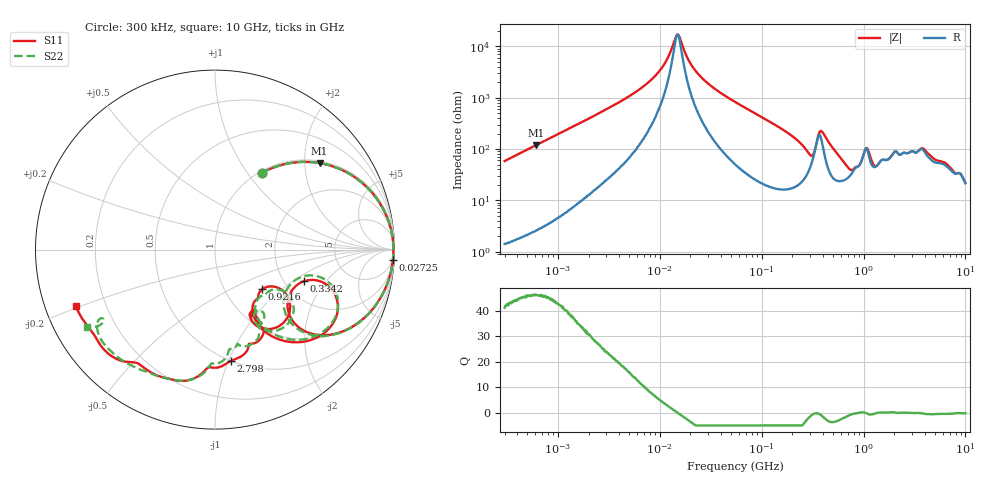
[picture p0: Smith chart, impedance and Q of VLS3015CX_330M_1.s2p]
! S-Parameter Data Generated by TDK Corporation
! Copyright(C) 2020 TDK Corporation.
! All Rights Reserved.
! TDK P/N: VLS3015CX-330M-1 (Inductor)
! Property: L=33uH at 1MHz
! Size(LxWxT): 3x3x1.5mm
! Model Type: s2p (Touchstone File Format Version 1.0)
! Frequency: DC=Yes Start=0.3MHz Stop=10000MHz 802points Log-sweep
! Model Generated on Aug. 18, 2020
! Port Assignments:
!  1 ---@@@--- 2
! Applicable Conditions:
!  Temperature = 25 degC
!  DC Bias Current = 0 A
!  Small Signal Operation
! Terms and conditions regarding TDK Simulation Models
! (1)This simulation model is being provided solely for informational purposes. Please refer to the specifications of the products in terms of detailed characteristics of such products.
! (2)In no event shall TDK Corporation of any of its subsidiaries be liable for any loss or damage arising, directly or indirectly,
!  From any information contained in this simulation model, including, but not limited to loss or damages arising from any inaccuracies, omissions or errors in connection with such information.
! (3)Any and all copyrights on this simulation model are owned by TDK Corporation.
!  Duplication or redistribution of this simulation model without prior written permission from TDK Corporation is prohibited.
! (4)This simulation model is subject to any modification or change without any prior notice.
! (5)Neither TDK Corporation nor any of its subsidiaries shall make any warranty, express or implied,
!  Including but not limited to the correctness, implied warranties of merchantability and fitness for a particular purpose with respect to this simulation models.
! (6)The use of this simulation model shall be deemed to have consented to the terms and conditions hereof.
# Hz S MA R 50
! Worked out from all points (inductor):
!   801 points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, 300 kHz to 10 GHz, reference 50 ohm
!   read as one part in series: L = 31 uH near 318.3 kHz
!   highest Q = 46.2 at 610.3 kHz (marker M1), where L = 30.9 uH
!   self-resonance near 14.9 MHz
!   S11 on the Smith chart (normalised r, x): 300 kHz: 1.03, +1.17; 27.25 MHz: 4, -34; 334.2 MHz: 2.53, -1.23; 921.6 MHz: 1.49, -0.75; 2.798 GHz: 0.50, -1.02; 10 GHz: 0.09, -0.19
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300000  0.4998 58.7  0.8544 -29.9  0.8538 -29.9  0.4991 58.7
610333  0.7562 39.6  0.6373 -49.2  0.6374 -49.1  0.7564 39.6
1713600  0.9499 16.5  0.285 -71.8  0.285 -71.8  0.9501 16.5
9671944  0.9937 1.5  0.03187 -78.1  0.03185 -78.1  0.9937 1.5
1.49005e7  0.9941 -0.4  0.005795 -3.4  0.005776 -3.5  0.9942 -0.4
2.036513e7  0.9938 -1.8  0.02258 73.3  0.02256 73.3  0.9938 -1.8
2.725275e7  0.9929 -3.3  0.04479 79.1  0.04477 79.1  0.9929 -3.3
5.477226e7  0.9856 -8.3  0.1184 78.2  0.1184 78.2  0.9857 -8.3
1.291483e8  0.9391 -20.6  0.296 66.1  0.2959 66.1  0.9389 -20.8
2.22675e8  0.7992 -36.4  0.5119 46.3  0.5118 46.3  0.7969 -36.9
3.126428e8  0.4887 -33.0  0.6014 10.8  0.6013 10.8  0.4644 -33.7
3.342219e8  0.525 -19.7  0.5036 0.8  0.5035 0.8  0.4974 -18.2
3.860116e8  0.7595 -25.7  0.3247 23.8  0.3247 23.8  0.7492 -23.5
4.986356e8  0.6871 -48.7  0.5795 28.5  0.5794 28.5  0.687 -47.0
6.987102e8  0.43 -59.9  0.7206 3.6  0.7205 3.6  0.4321 -57.6
9.216398e8  0.3437 -40.0  0.6474 -17.4  0.6472 -17.4  0.3824 -36.8
1.10164e9  0.5585 -46.5  0.4778 -9.6  0.4776 -9.6  0.5801 -46.8
1.276148e9  0.4314 -62.6  0.6345 -15.9  0.6344 -15.9  0.4443 -60.7
1.767019e9  0.4086 -60.5  0.5532 -37.6  0.5532 -37.6  0.492 -59.7
2.798208e9  0.6275 -82.0  0.4137 -51.9  0.4138 -51.9  0.577 -82.6
4.22443e9  0.7631 -108.8  0.3021 -56.0  0.3019 -56.0  0.7616 -108.0
1e10  0.8383 -157.8  0.2101 -86.9  0.2093 -86.9  0.8326 -148.9
